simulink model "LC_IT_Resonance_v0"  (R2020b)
settings: Solver=VariableStepAuto  StartTime=0.0  StopTime=2e-3  RelTol=1e-3
libraries: fl_lib x8, nesl_utility x3

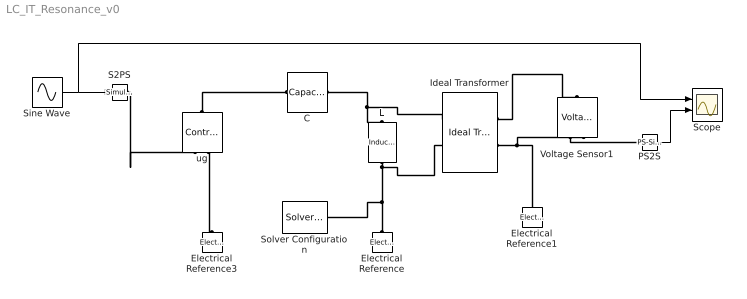
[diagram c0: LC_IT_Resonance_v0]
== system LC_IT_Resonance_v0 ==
  C : fl_lib/Electrical/Electrical Elements/Capacitor  c=1e-6 F  r=1e-6 Ohm  g=0 1/Ohm  i_specify=off  i_priority=None  i=0 A  i_nominal_specify=off  i_nominal_unit=A  i_nominal_value=1  v_specify=off  v_priority=None  v=0 V  v_nominal_specify=off  v_nominal_unit=V  v_nominal_value=1  vc_specify=off  vc_priority=High  vc=0 V  vc_nominal_specify=off  vc_nominal_unit=V  vc_nominal_value=1
  Electrical Reference : fl_lib/Electrical/Electrical Elements/Electrical Reference
  Electrical Reference1 : fl_lib/Electrical/Electrical Elements/Electrical Reference
  Electrical Reference3 : fl_lib/Electrical/Electrical Elements/Electrical Reference
  Ideal Transformer : fl_lib/Electrical/Electrical Elements/Ideal Transformer  n=1  i1_specify=off  i1_priority=None  i1=0 A  i1_nominal_specify=off  i1_nominal_unit=A  i1_nominal_value=1  v1_specify=off  v1_priority=None  v1=0 V  v1_nominal_specify=off  v1_nominal_unit=V  v1_nominal_value=1  i2_specify=off  i2_priority=None  i2=0 A  i2_nominal_specify=off  i2_nominal_unit=A  i2_nominal_value=1  v2_specify=off  v2_priority=None  v2=0 V  v2_nominal_specify=off  v2_nominal_unit=V  v2_nominal_value=1
  L : fl_lib/Electrical/Electrical Elements/Inductor  l=1e-4 H  r=0 Ohm  g=0 1/Ohm  i_specify=off  i_priority=None  i=0 A  i_nominal_specify=off  i_nominal_unit=A  i_nominal_value=1  v_specify=off  v_priority=None  v=0 V  v_nominal_specify=off  v_nominal_unit=V  v_nominal_value=1  i_L_specify=off  i_L_priority=High  i_L=0 A  i_L_nominal_specify=off  i_L_nominal_unit=A  i_L_nominal_value=1
  PS2S : nesl_utility/PS-Simulink Converter  PhysicalDomain=network_engine_domain  SubClassName=ps_output  LeftPortType=input  RightPortType=output  PseudoPeriodic=off  Frequencies=[]  Unit=inherit  AffineConversion=off
  S2PS : nesl_utility/Simulink-PS Converter  PhysicalDomain=network_engine_domain  SubClassName=ps_input  LeftPortType=input  RightPortType=output  PseudoPeriodic=off  Frequencies=[]  NoiseDistribution=none  NoiseParameters=[]  Unit=1  AffineConversion=off  FilteringAndDerivatives=provide  SimscapeFilterOrder=1  InputFilterTimeConstant=0.001  UdotUserProvided=0
  Scope : Scope  NumInputPorts=2
  Sine Wave : Sin  Frequency=1e5  SampleTime=0
  Solver Configuration : nesl_utility/Solver Configuration  PhysicalDomain=network_engine_domain  SubClassName=solver  LeftPortType=input  RightPortType=generic  Tones=[]  Harmonics=[]  SimulateNoise=off  Profile=off  UseLocalSampling=off  EnableSwitchedLinearOptims=on  FrequencyDomain=off  UseCCode=off  RelTol=0.001  AbsTol=1e-06  MinStep=1e-09  ToWorkspace=off  RevertToSquareIcSolve=off  NumHomotopyIterations=100  PhasorMode=off  PhasorModeNumHarmonics=1  DoDC=off  ResidualTolerance=1e-09  UseLocalSolver=off  LocalSolverChoice=NE_BACKWARD_EULER_ADVANCER  LocalSolverSampleTime=1e-5  DoFixedCost=off  MaxNonlinIter=3  MaxModeIter=2  ComputeImpulses=off  ImpulseIterations=2  LinearAlgebra=auto  EquationFormulation=NE_TIME_EF  DelaysMemoryBudget=1024  AutomaticFiltering=on  FilteringTimeConstant=1e-5  PartitionStorageMethod=AS_NEEDED  PartitionMemoryBudget=1024  PartitionMethod=ROBUST
  Voltage Sensor1 : fl_lib/Electrical/Electrical Sensors/Voltage Sensor
  ug : fl_lib/Electrical/Electrical Sources/Controlled Voltage Source
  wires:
  Sine Wave/1 -> Scope/1, S2PS/1
  PS2S/1 -> Scope/2
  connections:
  C/RConn1 -- Ideal Transformer/LConn1 -- L/LConn1
  L/RConn1 -- Solver Configuration/RConn1 -- Electrical Reference/LConn1 -- Ideal Transformer/LConn2
  ug/RConn2 -- Electrical Reference3/LConn1
  ug/LConn1 -- C/LConn1
  S2PS/RConn1 -- ug/RConn1
  Ideal Transformer/RConn2 -- Electrical Reference1/LConn1 -- Voltage Sensor1/RConn2
  Ideal Transformer/RConn1 -- Voltage Sensor1/LConn1
  Voltage Sensor1/RConn1 -- PS2S/LConn1
